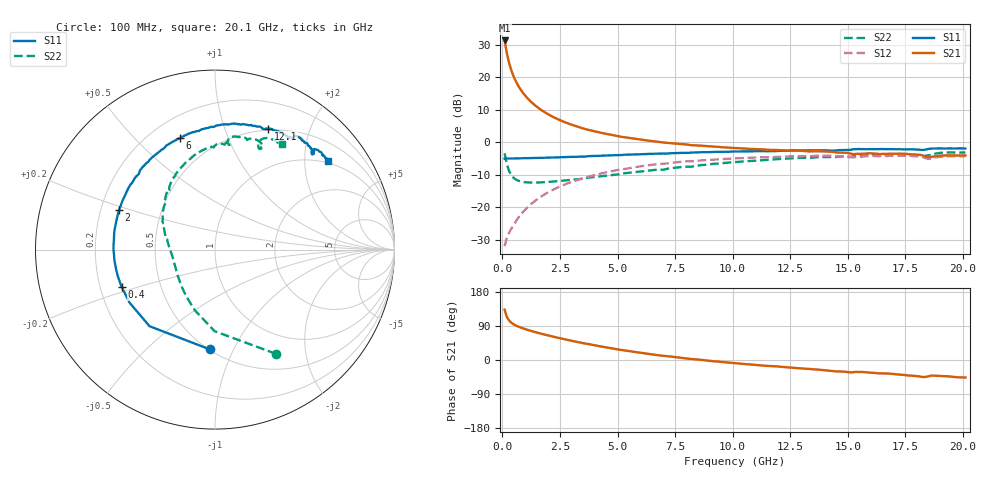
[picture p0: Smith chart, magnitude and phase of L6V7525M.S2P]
!  Infineon Technologies AG
! BFR380L3 , PF131585-7, No.6, Th 09.10.01, soldered on pcb-board, measured with PP GSG850
!  Vce=0.75 V,  Ic=25.0 mA
! Common Emitter S-Parameters:  15. November 2001
#  GHz  S  MA  R  50
! f  S11  S21  S12  S22
! GHz  Mag  Ang  Mag  Ang  Mag  Ang  Mag  Ang
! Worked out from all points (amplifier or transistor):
!   201 points, 100 MHz to 20.1 GHz, reference 50 ohm
!   highest |S21| = 31.3 dB at 100 MHz (marker M1)
!   |S21| within 3 dB of that: start of sweep to 173.7 MHz
!   unconditionally stable (mu >= 1): 1.114 GHz to 4.971 GHz; 5.167 GHz to 5.216 GHz; 18.31 GHz to 18.51 GHz
!   at 3.4 GHz: K = 1.02, MAG = 6.9 dB, |S12| = -11.3 dB
!   at 10.1 GHz: K = 0.98, MSG = 1.6 dB, |S12| = -5.0 dB
!   at 20.1 GHz: K = 0.99, MSG = 0.1 dB, |S12| = -4.3 dB
!   S11 on the Smith chart (normalised r, x): 100 MHz: 0.50, -0.81; 400 MHz: 0.29, -0.18; 2 GHz: 0.28, +0.18; 6 GHz: 0.32, +0.68; 12.1 GHz: 0.48, +1.42; 20.1 GHz: 0.95, +2.58
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0.1  0.5565 -93.0  36.78 132.8  0.02505 56.7  0.673 -59.6
0.2  0.5615 -130.5  23.02 113.0  0.03395 52.1  0.4549 -90.2
0.3  0.56 -147.9  16.26 103.8  0.04076 53.3  0.356 -108.4
0.4  0.5605 -158.0  12.49 98.0  0.0472 55.7  0.3071 -121.2
0.5  0.5614 -164.5  10.11 93.9  0.05408 58.3  0.2805 -130.6
0.6  0.562 -169.8  8.47 90.7  0.06152 60.1  0.2647 -137.9
0.7  0.5634 -173.9  7.308 87.9  0.06892 61.6  0.2549 -143.7
0.8  0.5633 -177.1  6.418 85.5  0.0766 62.6  0.2484 -148.5
0.9  0.5658 179.8  5.724 83.3  0.08425 63.4  0.244 -152.5
1.1  0.5656 174.8  4.719 79.4  0.09978 64.1  0.2402 -158.8
1.3  0.5696 170.4  4.017 75.7  0.1154 64.3  0.2386 -163.8
1.6  0.5722 164.5  3.295 70.8  0.1389 63.7  0.2398 -169.4
2  0.5787 157.6  2.674 64.7  0.1697 61.9  0.2441 -175.5
2.6  0.5861 148.4  2.106 56.2  0.2148 58.4  0.2547 177.2
3.5  0.598 135.7  1.63 44.5  0.2793 52.1  0.2715 168.2
6  0.6508 107.6  1.096 19.0  0.4238 33.9  0.3546 145.0
6.8  0.6655 100.1  1.01 12.4  0.4606 27.9  0.3768 137.4
10.1  0.717 76.3  0.8128 -8.2  0.5621 6.7  0.4935 112.8
12.1  0.7361 66.3  0.75 -18.0  0.5988 -4.8  0.5516 98.7
13.5  0.7467 59.6  0.7258 -24.6  0.6128 -12.7  0.5794 90.0
16.8  0.7793 47.7  0.6634 -35.9  0.6141 -27.5  0.6497 72.0
20.1  0.7987 38.2  0.6271 -46.2  0.6065 -40.4  0.695 57.5
